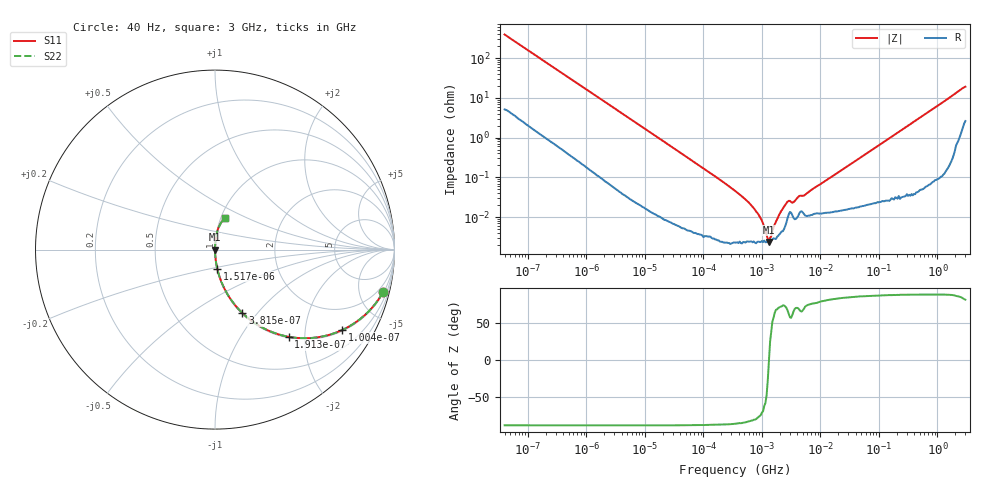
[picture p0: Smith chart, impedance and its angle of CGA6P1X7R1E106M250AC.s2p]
! S-parameter Generated by TDK Corporation
! Copyright(C) 2015 TDK Corporation.
! All Rights Reserved.
! TDK P/N: CGA6P1X7R1E106M250AC (Multilayer Ceramic Chip Capacitors)
! Property: C=10uF
! Size(LxWxT): 3.2x2.5x2.5mm, 0.126x0.098x0.098inches
! Model Type: s2p (Touchstone File Format Version 1.0)
! Frequency: DC=Yes Start=0.00004MHz Stop=3000MHz 396points Log-sweep
! Note: This model was converted from impedance.
! Model Generated on Jun. 23, 2015
! Hash(MD5):
! Port Assignments:
!  1 ---| |--- 2
! Applicable Conditions:
!  Temperature = 25 degC
!  DC Bias Voltage = 0 V
!  Small Signal Operation
! Terms and conditions regarding TDK Simulation Models
! (1)This simulation model is being provided solely for informational purposes. Please refer to the specifications of the products in terms of detailed characteristics of such products.
! (2)In no event shall TDK Corporation of any of its subsidiaries be liable for any loss or damage arising, directly or indirectly,
!  From any information contained in this simulation model, including, but not limited to loss or damages arising from any inaccuracies, omissions or errors in connection with such information.
! (3)Any and all copyrights on this simulation model are owned by TDK Corporation.
!  Duplication or redistribution of this simulation model without prior written permission from TDK Corporation is prohibited.
! (4)This simulation model is subject to any modification or change without any prior notice.
! (5)Neither TDK Corporation nor any of its subsidiaries shall make any warranty, express or implied,
!  Including but not limited to the correctness, implied warranties of merchantability and fitness for a particular purpose with respect to this simulation models.
! (6)The use of this simulation model shall be deemed to have consented to the terms and conditions hereof.
# MHz S MA R 50
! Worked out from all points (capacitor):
!   395 points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, 40 Hz to 3 GHz, reference 50 ohm
!   read as one part in series: C = 10.2 uF near 41.88 Hz
!   lowest |Z| = 2.39 mohm at 1.316 MHz (marker M1)
!   series resonance near 1.321 MHz, so ESL is about 1.4 nH
!   S11 on the Smith chart (normalised r, x): 40 Hz: 1.10, -7.85; 100.4 Hz: 1.04, -3.15; 191.3 Hz: 1.02, -1.66; 381.5 Hz: 1.01, -0.84; 1.517 kHz: 1.00, -0.22; 3 GHz: 1.05, +0.38
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4e-05  0.966 -14.3  0.2462 75.0  0.2462 75.0  0.966 -14.3
6.63624e-05  0.917 -22.8  0.387 66.5  0.387 66.5  0.917 -22.8
0.0001004175  0.8393 -32.2  0.5331 57.1  0.5331 57.1  0.8393 -32.2
0.0001912643  0.6357 -49.8  0.7641 39.5  0.7641 39.5  0.6357 -49.8
0.0003814572  0.3857 -66.6  0.918 22.7  0.918 22.7  0.3857 -66.6
0.000834128  0.1902 -78.4  0.9796 11.0  0.9796 11.0  0.1902 -78.4
0.001517294  0.107 -83.3  0.9932 6.1  0.9932 6.1  0.107 -83.3
0.004176322  0.03963 -87.2  0.9988 2.3  0.9988 2.3  0.03963 -87.2
0.01739424  0.009631 -88.8  0.9998 0.6  0.9998 0.6  0.009631 -88.8
0.3464102  0.0004591 -87.1  1 0.0  1 0.0  0.0004591 -87.1
0.6017834  0.0002294 -84.0  1 0.0  1 0.0  0.0002294 -84.0
0.9105995  0.0001043 -76.8  1 0.0  1 0.0  0.0001043 -76.8
1.315913  2.386e-05 -2.8  1 0.0  1 0.0  2.386e-05 -2.8
1.901634  0.0001038 70.8  1 -0.0  1 -0.0  0.0001038 70.8
2.748062  0.0002459 67.2  0.9999 -0.0  0.9999 -0.0  0.0002459 67.2
3.459106  0.0002368 65.9  0.9999 -0.0  0.9999 -0.0  0.0002368 65.9
4.354128  0.0003407 68.5  0.9999 -0.0  0.9999 -0.0  0.0003407 68.5
5.234209  0.0003499 69.9  0.9999 -0.0  0.9999 -0.0  0.0003499 69.9
7.22376  0.0004994 76.8  0.9999 -0.0  0.9999 -0.0  0.0004994 76.8
150.6385  0.00965 87.9  0.9997 -0.6  0.9997 -0.6  0.00965 87.9
906.6656  0.05686 85.9  0.9975 -3.3  0.9975 -3.3  0.05686 85.9
3000  0.1831 71.7  0.9584 -10.4  0.9584 -10.4  0.1831 71.7
